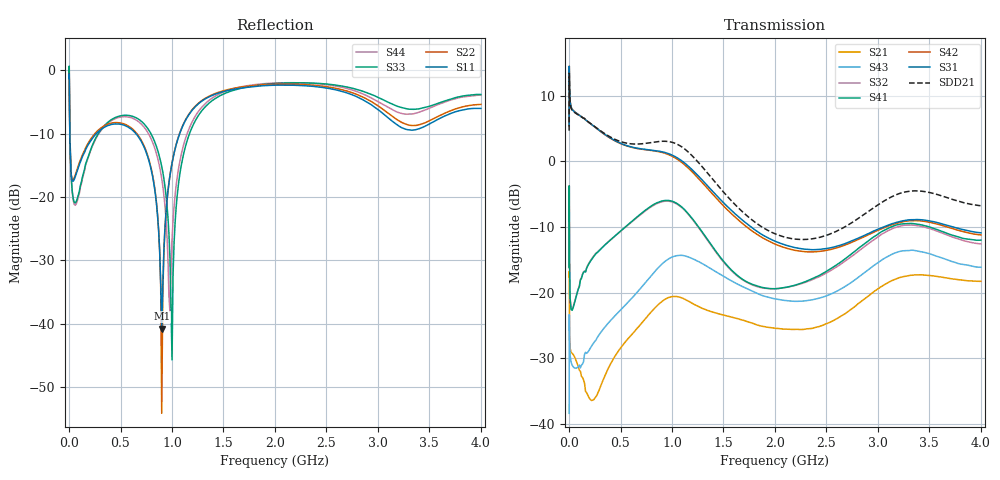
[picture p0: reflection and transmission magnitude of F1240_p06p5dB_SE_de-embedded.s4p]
! Integrated Device Technology
! Corporate Headquarters
! 6024 Silver Creek Valley Road
! San Jose, CA 95138  USA
! Phone:  1-408-284-8200
! Toll Free:  1-800-223-1366
! Webpage:  http://www.idt.com/
! Timing and RF Division
! 515 Groton Road, Suite 102
! Westford, MA 01886-6024
! Device:  F1240
! Description: Dual Intermediate Frequency Digital Variable Gain Amplifier
! Frequency:  10.0 -  500.00 MHz
! Package:  5x5 mm QFN Plastic Package: 32 pin
! Ports:  8 RF, 20 DC
!  Pin  1  = GA3 / Data  Pin 17  = RF OUT_B+
!  Pin  2  = GA4 / CLK  Pin 18  = RF OUT_B-
!  Pin  3  = GA5  Pin 19  = STBY_B
!  Pin  4  = VMODE  Pin 20  = Ground
!  Pin  5  = No Connect  Pin 21  = Ground
!  Pin  6  = GB5  Pin 22  = STB_A
!  Pin  7  = GB4  Pin 23  = RF OUT_A-  = Port 4
!  Pin  8  = GB3  Pin 24  = RF OUT_A+  = Port 3
!  Pin  9  = GB2  Pin 25  = GA0
!  Pin 10  = GB1  Pin 26  = ISET_A
!  Pin 11  = RF IN_B+  Pin 27  = VCC
!  Pin 12  = RF IN_B-  Pin 28  = Ground
!  Pin 13  = Ground  Pin 29  = RF IN_A-  = Port 2
!  Pin 14  = VCC  Pin 30  = RF IN_A+  = Port 1
!  Pin 15  = ISET_B  Pin 31  = GA1
!  Pin 16  = GB0  Pin 32  = GA2 / CSb
! Gain  = +19.5 dB
! State  = 1
! Voltage  = +5.00 V
! Current  = 85.292 mA (one channel only)
! Temperture  =  +25 C
! Test Date  =  2017-10-18
! Board  =  EB4031
! Data:  The device was measured on a custom evaluation board which has
!  individual transmission lines to the RF pins.  Data was collected
!  using a calibrated network analyzer.  The evaluation board was
!  de-embedded using Automatic Fixture Removal.
!  The reference plane is the edge of the package pin.
!  Only Channel A was measured.
!  This data is in single-ended operation.  If your needs are balanced
!  or differential S-parameters then this file needs to be used a
!  linear simulator.
! File Date:  2017-11-10  MJV
! Note:
!  Integrated Device Technology supplies this data as a sample of measured
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# Hz S dB R 100
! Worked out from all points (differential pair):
!   410 points, 500 kHz to 4 GHz, reference 100 ohm
!   strongest paths, dB at 500 kHz, 930 MHz, 1.96 GHz, 2.98 GHz, 4 GHz:
!     S31: 5.5, 1.4, -11.9, -10.5, -10.9
!     S42: 5.4, 1.2, -12.3, -10.6, -11.2
!     S41: -16.1, -5.9, -19.4, -11.3, -12.0
!     S32: -16.2, -6.1, -19.4, -11.7, -12.6
!     S43: -38.4, -15.2, -20.8, -15.6, -16.1
!     S21: -17.6, -21.0, -25.3, -19.6, -18.3
!   taken as a pair (ports 1,2 in; 3,4 out), SDD21 dB: 4.7, 3.1, -10.7, -6.8, -6.7
!   lowest |S11| = -40.8 dB at 900 MHz (marker M1), VSWR 1.02, Z = 98.4 - j0.747 ohm
!   |S11| at or under -10 dB: 7.491 MHz to 263.3 MHz (255.8 MHz wide, 189 % of centre); 650 MHz to 1.074 GHz (424.3 MHz wide, 49.2 % of centre)
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500000  -1.19 -5.5  -17.56 -5.7  -27.57 82.7  -49.58 78.0
        -17.56 -5.7  -1.19 -5.5  -49.60 76.7  -27.57 83.9
        5.45 -105.3  -16.19 -99.3  -0.46 1.4  -38.42 -83.1
        -16.12 -98.2  5.43 -104.1  -38.36 -83.1  -0.47 3.7
3000000  -3.49 -59.4  -22.71 -60.6  -15.94 26.0  -42.26 -11.0
         -22.74 -60.4  -3.45 -59.4  -42.18 -11.3  -15.95 26.2
         13.55 176.7  -8.06 148.0  -1.85 -58.8  -24.10 -171.0
         -8.16 147.9  13.55 176.9  -24.06 -171.0  -1.90 -58.6
3e7  -17.45 -102.9  -29.18 -18.4  -16.30 -8.0  -45.40 20.1
     -29.21 -18.4  -17.25 -103.2  -45.36 20.6  -16.29 -7.9
     7.93 161.9  -22.54 109.5  -18.96 -124.7  -31.15 156.4
     -22.66 109.9  7.96 161.9  -31.02 156.6  -19.17 -125.3
1.9e8  -11.63 -134.9  -35.85 -31.1  -17.76 -48.3  -35.66 17.7
       -35.86 -29.7  -11.35 -135.8  -35.65 18.4  -17.78 -48.5
       5.98 112.2  -15.56 22.3  -13.39 -116.8  -29.11 98.7
       -15.65 22.2  5.97 111.5  -28.86 98.2  -13.52 -115.8
5.2e8  -8.57 -178.1  -28.38 -25.2  -18.90 -109.3  -29.83 -56.0
       -28.01 -25.5  -8.38 -179.5  -29.94 -53.8  -19.02 -109.6
       2.64 26.6  -10.38 -66.5  -7.11 -164.2  -22.80 9.4
       -10.34 -67.7  2.59 25.7  -22.31 9.1  -7.32 -164.3
9e8  -40.79 -155.4  -21.56 -95.9  -17.30 166.6  -27.05 -142.1
     -21.35 -100.0  -54.20 119.0  -27.19 -135.5  -17.60 165.6
     1.48 -69.7  -6.15 -178.5  -15.17 134.3  -16.19 -79.7
     -6.04 178.2  1.39 -71.6  -15.66 -81.1  -17.10 136.4
4e9  -6.00 -144.2  -18.33 94.3  -21.95 -66.3  -22.97 -46.7
     -18.26 93.7  -5.36 -142.9  -23.81 -28.8  -23.48 -60.3
     -10.87 21.7  -12.56 -91.2  -3.79 -138.6  -17.14 75.5
     -11.99 -105.4  -11.19 28.2  -16.12 58.9  -3.90 -147.0
